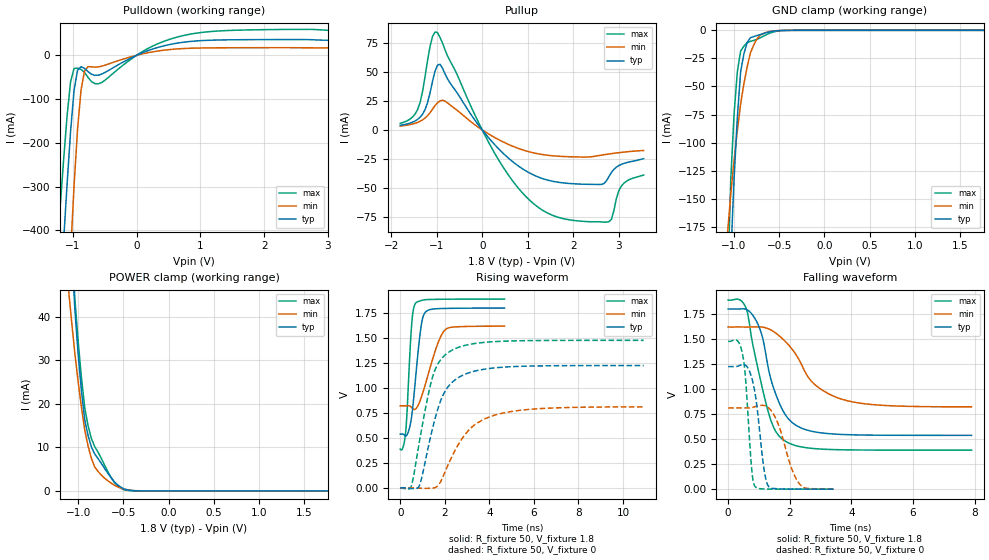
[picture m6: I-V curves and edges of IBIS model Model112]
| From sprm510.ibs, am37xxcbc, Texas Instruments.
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| Model based on original model for BQ18OMAPSMART2HYFBPB_SSBHH
|   Sub model HYFBPB_H_0_PUPD0_1P8
[model]   Model112
|[Input Load]   PI
|[Output Drive] LB0
|Voltage   1.8V
|Mode   I/O
Model_type   I/O
Polarity   Non-Inverting
Enable   Active-Low
Vinl =  0.63
Vinh =  1.17
Cref =  15pF
Rref =  100.0000M
Vref =  0V
Vmeas =  0.9
C_comp   1.528652p   1.368776p   1.69933p
[Model Spec]
Vinl   0.63   0.567   0.6615
Vinh   1.17   1.053   1.2285
[Temperature Range]   25   125   -40
[Voltage Range]   1.8   1.62   1.89
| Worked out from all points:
|   slope of the pulldown table from 0 to 0.27 V, typ, clamps not added: 17.8 ohm
|   slope of the pullup table from 0 to 0.27 V, typ, clamps not added: 21.5 ohm
|   GND clamp passes 1 mA (typ) near -0.58 V on its own axis
|   POWER clamp passes 1 mA (typ) near -0.54 V on its own axis
|   rising waveform, R_fixture 50, V_fixture 1.8: 20-80 % time 341ps typ, 657ps min, 211ps max; typ from 0.538 V to 1.8 V
|   rising waveform, R_fixture 50, V_fixture 0: 20-80 % time 943ps typ, 1.43ns min, 829ps max; typ from 0 V to 1.22 V
|   falling waveform, R_fixture 50, V_fixture 1.8: 20-80 % time 681ps typ, 1.19ns min, 663ps max; typ from 1.8 V to 0.538 V
|   falling waveform, R_fixture 50, V_fixture 0: 20-80 % time 281ps typ, 490ps min, 196ps max; typ from 1.22 V to 0 V
[POWER_clamp]
-1.8V     449.2mA    229.3mA    499.9mA
-1.109V   70.03mA    46.65mA    71.76mA
-1.073V   55.15mA    38.86mA    56.96mA
-1.036V   41.47mA    31.41mA    43.93mA
-1V       31.2mA     24.93mA    34.21mA
-963.6mV  22.8mA     19.1mA     25.91mA
-927.3mV  16.27mA    13.92mA    19.01mA
-890.9mV  12.72mA    10.32mA    14.97mA
-818.2mV  8.506mA    5.529mA    10.22mA
-600mV    2.086mA    1.321mA    1.925mA
-381.8mV  46uA       75.05uA    15.45uA
1.764V    -1.701nA   -102nA     -1.875nA
[Pulldown]
-1.8V     -1.866A    -2.926A    -1.473A
-1.255V   -690.3mA   -1.165A    -458.8mA
-1.2V     -556.9mA   -981.3mA   -347.5mA
-1.145V   -424mA     -799.3mA   -238.7mA
-1.036V   -174.1mA   -452.5mA   -60.31mA
-981.8mV  -80.13mA   -298.3mA   -30.04mA
-872.7mV  -26.27mA   -79.78mA   -32.44mA
-763.6mV  -37.26mA   -25.87mA   -50.47mA
-545.5mV  -42.85mA   -24.82mA   -62.02mA
163.6mV   9.905mA    5.464mA    14.49mA
872.7mV   32.06mA    16.22mA    49.12mA
3.545V    34.18mA    16.99mA    56.07mA
[Pullup]
-1.8V     4.02mA     3.353mA    5.71mA
-1.418V   9.153mA    6.524mA    17.71mA
-1.255V   17.65mA    10.28mA    46.45mA
-1.091V   42.12mA    17.99mA    80.97mA
-981.8mV  56.04mA    23.5mA     84.34mA
-818.2mV  48.72mA    25.01mA    69.63mA
272.7mV   -12.68mA   -6.535mA   -20.08mA
1.255V    -41.13mA   -20.87mA   -67.69mA
2.564V    -47.26mA   -22.22mA   -79.57mA
2.782V    -40.42mA   -20.82mA   -79.47mA
3.055V    -29.85mA   -19.43mA   -48.72mA
3.545V    -24.9mA    -17.8mA    -39.06mA
[GND_clamp]
-1.8V     -3.26A     -1.496A    -3.636A
-1.073V   -295.4mA   -181.3mA   -234.2mA
-1.036V   -202.1mA   -145.8mA   -132.5mA
-1V       -132.6mA   -116.1mA   -74.83mA
-963.6mV  -77.56mA   -89.36mA   -36.83mA
-927.3mV  -36.94mA   -65.52mA   -18.53mA
-890.9mV  -20.86mA   -47.5mA    -14.02mA
-854.5mV  -10.73mA   -32.34mA   -11.09mA
-818.2mV  -6.545mA   -20.02mA   -9.764mA
-709.1mV  -3.764mA   -4.146mA   -6.62mA
-563.6mV  -769uA     -544.8uA   -1.476mA
1.764V    -87.86pA   812.3nA    3.194nA
[Ramp]
dV/dt_f  0.7587808/0.681029n   0.4797485/1.197896n   0.9054589/0.6658081n
dV/dt_r  0.7390206/0.9440878n  0.4899682/1.440888n   0.8942135/0.832063n
R_load = 50
[Rising Waveform]
R_fixture = 50
V_fixture = 1.8
V_fixture_min = 1.62
V_fixture_max = 1.89
0s        537.7mV    821mV      387.2mV
126ps     537.8mV    821.3mV    408mV
243ps     518mV      820.9mV    556.2mV
504ps     702.5mV    805.3mV    1.61V
684ps     1.088V     788.3mV    1.847V
963ps     1.654V     917.1mV    1.876V
1.17ns    1.766V     1.07V      1.884V
1.701ns   1.794V     1.454V     1.887V
2.07ns    1.796V     1.592V     1.888V
4.68ns    1.799V     1.618V     1.89V
[Rising Waveform]
R_fixture = 50
V_fixture = 0
V_fixture_min = 0
V_fixture_max = 0
0s        -338.8uV   73.66uV    -1.181mV
450ps     -5.934mV   1.362mV    -5.958mV
585ps     -7.232mV   -38.87uV   99.48mV
837ps     10.36mV    -3.219mV   432.5mV
1.485ns   625.6mV    -2.172mV   1.134V
1.863ns   899.1mV    84.72mV    1.295V
2.241ns   1.036V     276.1mV    1.367V
3.159ns   1.157V     595.9mV    1.438V
4.374ns   1.204V     736.1mV    1.465V
10.93ns   1.224V     809.9mV    1.477V
[Falling Waveform]
R_fixture = 50
V_fixture = 1.8
V_fixture_min = 1.62
V_fixture_max = 1.89
0s        1.8V       1.62V      1.89V
351ps     1.8V       1.62V      1.895V
576ps     1.798V     1.62V      1.813V
918ps     1.678V     1.621V     1.273V
1.116ns   1.516V     1.619V     1.001V
1.413ns   1.07V      1.586V     664.9mV
1.89ns    728.7mV    1.465V     472.7mV
2.754ns   575.8mV    1.062V     406.6mV
3.69ns    546.6mV    898.3mV    393.5mV
7.902ns   537.9mV    822.7mV    390.2mV
[Falling Waveform]
R_fixture = 50
V_fixture = 0
V_fixture_min = 0
V_fixture_max = 0
0s        1.224V     811.6mV    1.476V
306ps     1.228V     811.9mV    1.482V
486ps     1.245V     811.7mV    1.318V
576ps     1.235V     811.4mV    1.061V
765ps     1.113V     815.1mV    197.6mV
873ps     960.2mV    824.2mV    27.52mV
1.179ns   170mV      835mV      1.64mV
1.332ns   18.32mV    806.9mV    984.9uV
2.322ns   478.4uV    49.9mV     212.4uV
3.42ns    123.7uV    1.651mV    50.78uV
